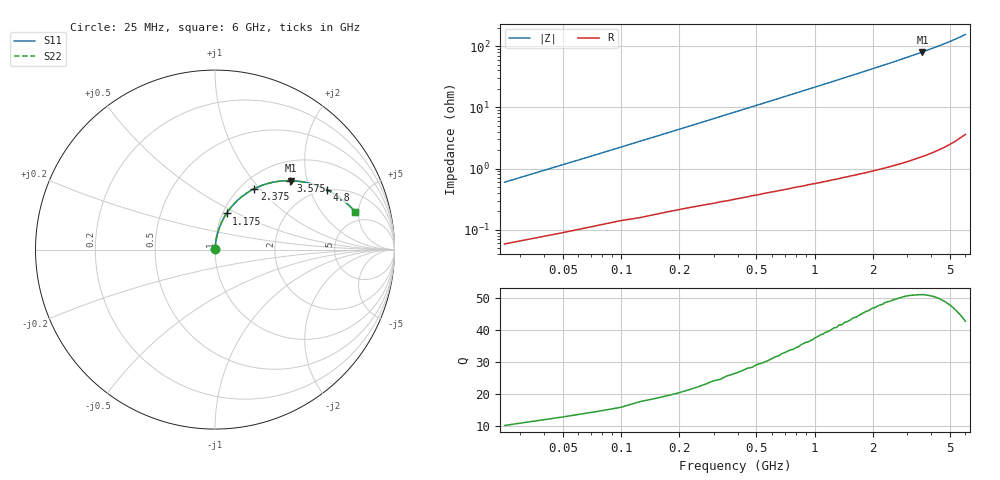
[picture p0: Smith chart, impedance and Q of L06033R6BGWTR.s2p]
!	AVX Thin Film Operation
!	Date:	March	2003
!	Description: Accu-L® Series Thin Film SMD RF Inductors
!	Part Number: L06033R6BGWTR
!	25MHz-6GHz
!	Serial	Measurements
#	mhz	S	db	R	50
!	S11	S11	S21	S21	S12	S12	S22	S22
!	dB	Phase	dB	Phase	dB	Phase	dB	Phase
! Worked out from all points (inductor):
!   240 points, 25 MHz to 6 GHz, reference 50 ohm
!   read as one part in series: L = 3.6 nH near 50 MHz
!   highest Q = 51.2 at 3.6 GHz (marker M1), where L = 3.54 nH
!   S11 on the Smith chart (normalised r, x): 25 MHz: 1.00, +0.01; 1.175 GHz: 1.04, +0.44; 2.375 GHz: 1.16, +0.94; 3.575 GHz: 1.40, +1.59; 4.8 GHz: 1.97, +2.62; 6 GHz: 3.78, +4.59
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25  -45.56 83.0  -0.01 -0.4  -0.01 -0.4  -45.56 83.0
50  -39.90 84.0  -0.01 -0.7  -0.01 -0.7  -39.90 84.0
75  -36.55 84.4  -0.01 -1.1  -0.01 -1.1  -36.55 84.4
100  -34.16 84.5  -0.01 -1.4  -0.01 -1.4  -34.16 84.5
125  -32.30 84.4  -0.02 -1.8  -0.02 -1.8  -32.30 84.4
175  -29.49 84.2  -0.02 -2.5  -0.02 -2.5  -29.49 84.2
275  -25.69 83.3  -0.03 -3.9  -0.03 -3.9  -25.69 83.3
400  -22.54 82.0  -0.05 -5.6  -0.05 -5.6  -22.54 82.0
575  -19.48 79.9  -0.08 -7.9  -0.08 -7.9  -19.48 79.9
775  -16.97 77.4  -0.13 -10.6  -0.13 -10.6  -16.97 77.4
1025  -14.63 74.2  -0.20 -14.0  -0.20 -14.0  -14.63 74.2
1175  -13.50 72.3  -0.25 -16.0  -0.25 -16.0  -13.50 72.3
1575  -11.10 67.2  -0.41 -21.3  -0.41 -21.3  -11.10 67.2
2025  -9.09 61.5  -0.65 -27.1  -0.65 -27.1  -9.09 61.5
2375  -7.86 57.1  -0.86 -31.5  -0.86 -31.5  -7.86 57.1
3025  -6.06 49.0  -1.34 -39.6  -1.34 -39.6  -6.06 49.0
3575  -4.89 42.4  -1.82 -46.2  -1.82 -46.2  -4.89 42.4
3600  -4.85 42.1  -1.85 -46.5  -1.85 -46.5  -4.85 42.1
4025  -4.11 37.1  -2.27 -51.5  -2.27 -51.5  -4.11 37.1
4800  -3.03 28.3  -3.16 -60.4  -3.16 -60.4  -3.03 28.3
5025  -2.77 25.7  -3.45 -62.9  -3.45 -62.9  -2.77 25.7
6000  -1.83 15.0  -4.89 -73.5  -4.89 -73.5  -1.83 15.0
